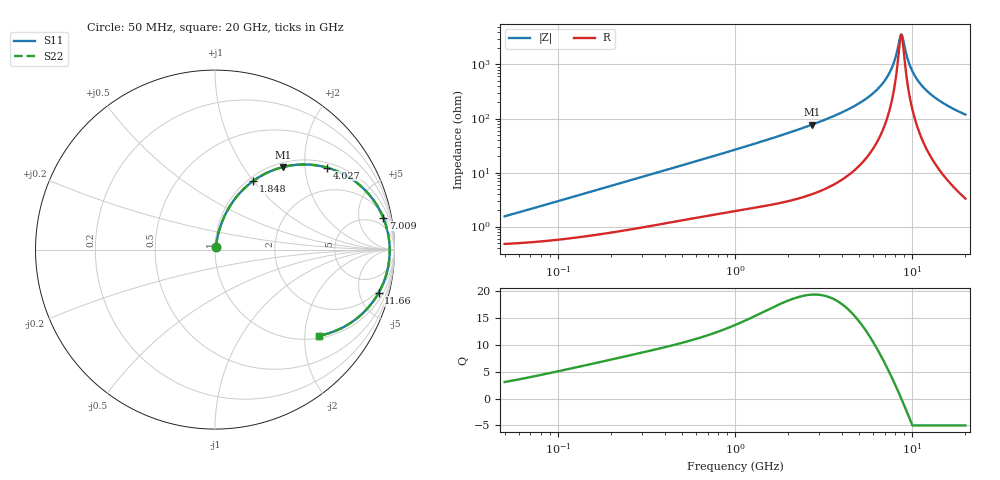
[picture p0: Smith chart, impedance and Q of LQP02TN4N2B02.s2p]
!Murata Part Number: LQP02TN4N2B02
!These Parameters are Measured in Series Mode Connection
!  o--[Z]--o
!Port1  Port2
!  o-------o
!Freq. Start=50[MHz] Stop=20[GHz], 401[Steps]
# Hz S RI R 50
!Freq.(Hz) S11(Real) S11(Imag) S21(Real) S21(Imag) S12(Real) S12(Imag) S22(Real) S22(Imag)
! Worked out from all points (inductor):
!   401 points, 50 MHz to 20 GHz, reference 50 ohm
!   read as one part in series: L = 4.67 nH near 51.52 MHz
!   highest Q = 19.4 at 2.728 GHz (marker M1), where L = 4.5 nH
!   self-resonance near 8.645 GHz
!   S11 on the Smith chart (normalised r, x): 50 MHz: 1.01, +0.03; 1.848 GHz: 1.06, +0.99; 4.027 GHz: 1.15, +2.60; 7.009 GHz: 3, +10; 11.66 GHz: 1.69, -7.34; 20 GHz: 1.07, -2.36
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5e7  0.00497 0.0146  0.995 -0.0146  0.995 -0.0146  0.00497 0.0146
1.364002e8  0.00791 0.0385  0.9921 -0.0385  0.9921 -0.0385  0.00791 0.0385
3.721004e8  0.0207 0.0985  0.9793 -0.0985  0.9793 -0.0985  0.0207 0.0985
1e9  0.0807 0.2382  0.9193 -0.2382  0.9193 -0.2382  0.0807 0.2382
1.848039e9  0.2108 0.3807  0.7892 -0.3807  0.7892 -0.3807  0.2108 0.3807
2.728004e9  0.3793 0.4601  0.6207 -0.4601  0.6207 -0.4601  0.3793 0.4601
4.026975e9  0.6225 0.4571  0.3775 -0.4571  0.3775 -0.4571  0.6225 0.4571
5.598765e9  0.8352 0.3323  0.1648 -0.3323  0.1648 -0.3323  0.8352 0.3323
6.311513e9  0.8963 0.2563  0.1037 -0.2563  0.1037 -0.2563  0.8963 0.2563
7.009217e9  0.937 0.1788  0.063 -0.1788  0.063 -0.1788  0.937 0.1788
7.442007e9  0.9538 0.131  0.0462 -0.131  0.0462 -0.131  0.9538 0.131
7.901521e9  0.9656 0.0814  0.0344 -0.0814  0.0344 -0.0814  0.9656 0.0814
8.516016e9  0.9729 0.0177  0.0271 -0.0177  0.0271 -0.0177  0.9729 0.0177
8.644534e9  0.9733 0.00483  0.0267 -0.00483  0.0267 -0.00483  0.9733 0.00483
8.774992e9  0.9734 -0.00803  0.0266 0.00803  0.0266 0.00803  0.9734 -0.00803
8.907419e9  0.9732 -0.0209  0.0268 0.0209  0.0268 0.0209  0.9732 -0.0209
9.457416e9  0.9687 -0.0721  0.0313 0.0721  0.0313 0.0721  0.9687 -0.0721
9.892087e9  0.9618 -0.11  0.0382 0.11  0.0382 0.11  0.9618 -0.11
1.066139e10  0.9438 -0.1713  0.0562 0.1713  0.0562 0.1713  0.9438 -0.1713
1.166392e10  0.912 -0.2404  0.088 0.2404  0.088 0.2404  0.912 -0.2404
1.460232e10  0.7935 -0.3807  0.2065 0.3807  0.2065 0.3807  0.7935 -0.3807
2e10  0.5805 -0.4797  0.4195 0.4797  0.4195 0.4797  0.5805 -0.4797
